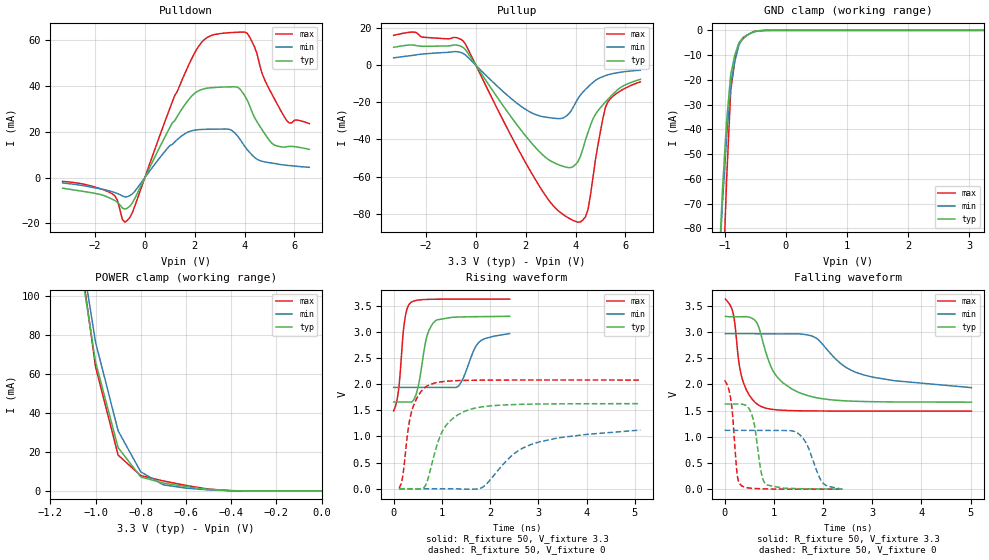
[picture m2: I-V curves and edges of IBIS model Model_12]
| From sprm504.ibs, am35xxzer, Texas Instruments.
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| Model based on original model for BC1833DV50BTPBFZP18LL_7LM
|   Sub model LL_7LM_PD_PU_OFF_3P3
[model]   Model_12
|[Description]  3.3V-I/O-PI-X
|[Input Load]   PI
|[Output Drive]
|Voltage   3.3V
|Mode   I/O
Model_type   I/O
Polarity   Non-Inverting
Enable   Active-Low
Vinl =  0.8V
Vinh =  2V
Cref =  15pF
Rref =  100.0000M
Vref =  0V
Vmeas =  1.65
C_comp   1.683006p   1.492615p   1.787227p
[Model Spec]
Vinl   0.8V   0.8V   0.8V
Vinh   2V   2V   2V
[Temperature Range]   25   125   -40
[Voltage Range]   3.3   2.97   3.63
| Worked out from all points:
|   slope of the pulldown table from 0 to 0.495 V, typ, clamps not added: 44.6 ohm
|   slope of the pullup table from 0 to 0.495 V, typ, clamps not added: 49.2 ohm
|   GND clamp passes 1 mA (typ) near -0.56 V on its own axis
|   POWER clamp passes 1 mA (typ) near -0.51 V on its own axis
|   rising waveform, R_fixture 50, V_fixture 3.3: 20-80 % time 193ps typ, 277ps min, 121ps max; typ from 1.66 V to 3.3 V
|   rising waveform, R_fixture 50, V_fixture 0: 20-80 % time 429ps typ, 980ps min, 234ps max; typ from 0 V to 1.63 V
|   falling waveform, R_fixture 50, V_fixture 3.3: 20-80 % time 517ps typ, 992ps min, 229ps max; typ from 3.3 V to 1.66 V
|   falling waveform, R_fixture 50, V_fixture 0: 20-80 % time 154ps typ, 283ps min, 108ps max; typ from 1.63 V to 0 V
[POWER_clamp]
-3.3V     2.414A     2.855A     2.597A
-1.067V   116.4mA    125.1mA    120.1mA
-1.033V   91.27mA    100.7mA    91.89mA
-1V       66.16mA    76.3mA     63.65mA
-900mV    22.18mA    30.79mA    18.35mA
-800mV    7.186mA    9.78mA     7.855mA
-700mV    3.999mA    3.101mA    5.133mA
-600mV    2.231mA    1.427mA    2.811mA
-500mV    830.8uA    532.6uA    931.1uA
-400mV    130.7uA    108.8uA    101.5uA
0V        9.334nA    42.91nA    36.63nA
[Pulldown]
-3.3V     -4.655mA   -2.337mA   -1.677mA
-1.3V     -9.504mA   -6.223mA   -7.163mA
-900mV    -13.3mA    -8.026mA   -18.36mA
-700mV    -13.35mA   -8.345mA   -18.7mA
1.8V      34.68mA    20.21mA    50.21mA
2.3V      38.61mA    21.07mA    59.44mA
2.8V      39.41mA    21.2mA     62.61mA
3.5V      39.7mA     20.55mA    63.45mA
4.1V      34.07mA    12.32mA    63.18mA
5V        16.21mA    6.501mA    38.53mA
5.7V      13.51mA    5.366mA    24.85mA
6.6V      12.35mA    4.495mA    23.63mA
[Pullup]
-3.3V     9.687mA    4.009mA    16.14mA
-2.5V     10.88mA    5.407mA    17.91mA
-500mV    9.486mA    6.336mA    12.94mA
1.4V      -27.6mA    -17.76mA   -37.69mA
2.4V      -44.47mA   -26.6mA    -61.92mA
3.5V      -54.49mA   -28.37mA   -80.48mA
4.1V      -51.87mA   -17.91mA   -84.62mA
4.5V      -36.09mA   -11.65mA   -77.77mA
4.8V      -26.39mA   -8.135mA   -50.71mA
5.2V      -19.78mA   -5.578mA   -22.57mA
5.6V      -14.26mA   -4.206mA   -15.61mA
6.6V      -7.577mA   -2.662mA   -8.942mA
[GND_clamp]
-3.3V     -1.975A    -1.766A    -3.378A
-1.1V     -99.4mA    -100.8mA   -162mA
-1.033V   -63.74mA   -69.32mA   -106.1mA
-966.7mV  -36.57mA   -43.05mA   -60.18mA
-900mV    -17.88mA   -22.01mA   -24.32mA
-833.3mV  -10mA      -12.38mA   -12.34mA
-766.7mV  -5.046mA   -6.023mA   -5.36mA
-700mV    -3.007mA   -2.937mA   -3.388mA
-566.7mV  -1.046mA   -1.097mA   -993.1uA
-500mV    -384.7uA   -514.4uA   -290.6uA
-300mV    -14.31uA   -22.54uA   -14.39uA
3.233V    8.947nA    10.19uA    33.58nA
[Ramp]
dV/dt_f 0.98336829/0.50708992n 0.61878131/0.98680858n  1.2831261/0.2283362n
dV/dt_r  0.9821883/0.4250305n 0.67877027/0.97564294n  1.2533892/0.23156395n
R_load = 50
[Rising Waveform]
R_fixture = 50
V_fixture = 3.3
V_fixture_min = 2.97
V_fixture_max = 3.63
538fs     1.661V     1.939V     1.491V
104.4ps   1.661V     1.939V     1.911V
227.6ps   1.661V     1.939V     3.212V
338.1ps   1.66V      1.939V     3.549V
471ps     1.821V     1.939V     3.605V
681.2ps   2.887V     1.939V     3.623V
863.1ps   3.211V     1.939V     3.627V
1.321ns   3.285V     1.948V     3.629V
1.76ns    3.294V     2.795V     3.63V
2.405ns   3.3V       2.97V      3.63V
[Rising Waveform]
R_fixture = 50
V_fixture = 0
V_fixture_min = 0
V_fixture_max = 0
115.4ps   8.191nV    109.8nV    4.108nV
188.1ps   4.844uV    -366.5nV   234.2mV
385.4ps   -3.782mV   -5.696nV   1.518V
626.8ps   22.11mV    144.5nV    1.919V
738.1ps   279.9mV    13.7nV     1.987V
1.025ns   1.125V     14.31uV    2.05V
1.488ns   1.488V     -6.912mV   2.074V
1.858ns   1.57V      36.68mV    2.078V
2.87ns    1.619V     853.6mV    2.081V
5.115ns   1.629V     1.123V     2.08V
[Falling Waveform]
R_fixture = 50
V_fixture = 3.3
V_fixture_min = 2.97
V_fixture_max = 3.63
15.96ps   3.3V       2.97V      3.63V
175.2ps   3.292V     2.97V      3.344V
297.2ps   3.291V     2.97V      2.368V
388.4ps   3.294V     2.97V      2.013V
613.4ps   3.225V     2.968V     1.662V
736.3ps   2.958V     2.966V     1.581V
1.042ns   2.173V     2.964V     1.516V
1.691ns   1.786V     2.944V     1.495V
2.71ns    1.677V     2.216V     1.492V
5.016ns   1.661V     1.939V     1.491V
[Falling Waveform]
R_fixture = 50
V_fixture = 0
V_fixture_min = 0
V_fixture_max = 0
0s        1.629V     1.123V     2.08V
117.3ps   1.625V     1.123V     1.748V
253.9ps   1.625V     1.123V     284.3mV
343.4ps   1.625V     1.123V     63.39mV
565.7ps   1.379V     1.122V     15.64mV
749.5ps   286.7mV    1.121V     7.079mV
853.3ps   81.2mV     1.121V     4.181mV
1.512ns   9.766mV    1.05V      160.3uV
1.988ns   3.806mV    127.7mV    20.6uV
2.395ns   8.191nV    109.8nV    4.108nV
